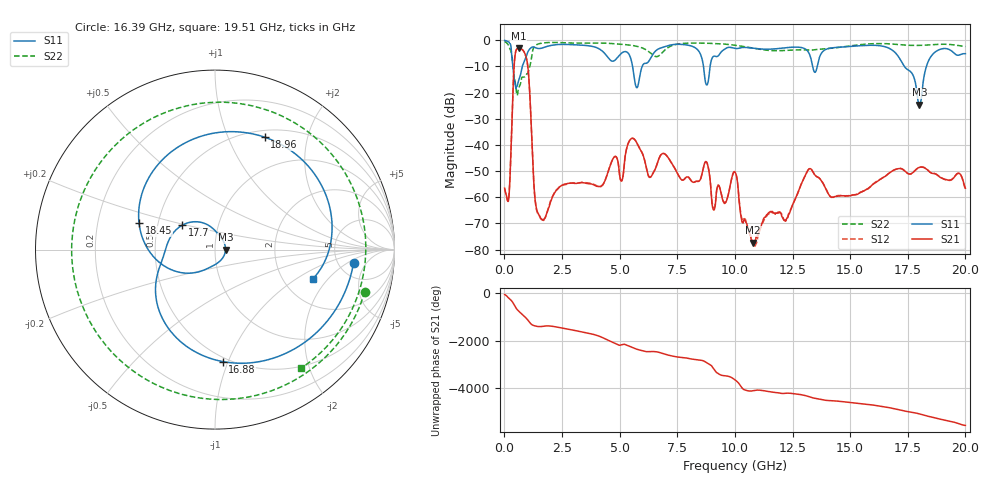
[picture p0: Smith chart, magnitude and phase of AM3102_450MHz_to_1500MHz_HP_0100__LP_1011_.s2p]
!Agilent Technologies,E8364B,MY43040894,A.07.50.67
!Agilent E8364B: A.07.50.67
!Date: Thursday, January 11, 2018 05:37:55
!Correction: S11(Full 2 Port(1,2))
!S21(Full 2 Port(1,2))
!S12(Full 2 Port(1,2))
!S22(Full 2 Port(1,2))
!S2P File: Measurements: S11, S21, S12, S22:
# Hz S  dB  R 50
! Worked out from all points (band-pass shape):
!   1601 points, 10 MHz to 20 GHz, reference 50 ohm
!   highest |S21| = -3.03 dB at 622.2 MHz (marker M1); lowest = -77.3 dB at 10.79 GHz (marker M2)
!   |S21| within 3 dB of the highest: 458.7 MHz to 929.5 MHz (470.8 MHz wide, 67.8 % of centre)
!   lowest |S11| = -24.6 dB at 18 GHz (marker M3), VSWR 1.12, Z = 56.2 - j0.0271 ohm
!   |S11| at or under -10 dB: 365.4 MHz to 775.7 MHz (410.3 MHz wide, 71.9 % of centre); 5.561 GHz to 5.976 GHz (415.1 MHz wide, 7.2 % of centre); 17.35 GHz to 18.31 GHz (952.8 MHz wide, 5.34 % of centre)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
!   |S22| runs from -21.0 to -0.5 dB; largest |S21 - S12| = 0.0025
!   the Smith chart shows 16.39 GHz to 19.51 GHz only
!   S11 on the Smith chart (normalised r, x): 16.39 GHz: 6.97, -2.54; 16.88 GHz: 0.47, -0.96; 17.7 GHz: 0.67, +0.19; 18.45 GHz: 0.39, +0.14; 18.96 GHz: 0.58, +1.37; 19.51 GHz: 2.89, -1.40
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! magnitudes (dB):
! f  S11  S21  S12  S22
! 10 MHz  -0.1  -56.5  -56.7  -0.5
! 184.9 MHz  -0.6  -60.8  -60.6  -2.1
! 447.3 MHz  -15.7  -7.0  -7.0  -14.7
! 622.2 MHz  -15.3  -3.0  -3.0  -18.2
! 997 MHz  -4.9  -8.7  -8.7  -12.7
! 1.484 GHz  -3.1  -66.6  -66.6  -1.4
! 3.346 GHz  -1.8  -54.3  -54.3  -1.1
! 5.745 GHz  -18.1  -39.2  -39.2  -2.3
! 6.682 GHz  -3.3  -45.7  -45.8  -6.0
! 9.08 GHz  -6.1  -64.9  -64.0  -1.2
! 10.01 GHz  -3.1  -50.4  -50.3  -1.9
! 10.79 GHz  -3.0  -77.3  -78.1  -3.0
! 13.34 GHz  -8.6  -49.6  -49.6  -3.7
! 16.39 GHz  -2.2  -52.7  -52.6  -1.2
! 16.68 GHz  -3.0  -50.9  -50.8  -1.3
! 16.88 GHz  -4.1  -49.7  -49.6  -1.5
! 17.7 GHz  -12.9  -50.7  -50.7  -1.9
! 18 GHz  -24.6  -48.6  -48.6  -1.9
! 18.45 GHz  -7.0  -50.3  -50.3  -1.7
! 18.96 GHz  -3.3  -52.6  -52.5  -1.5
! 19.51 GHz  -4.9  -52.3  -52.2  -1.8
! 20 GHz  -5.1  -56.5  -57.0  -2.4
